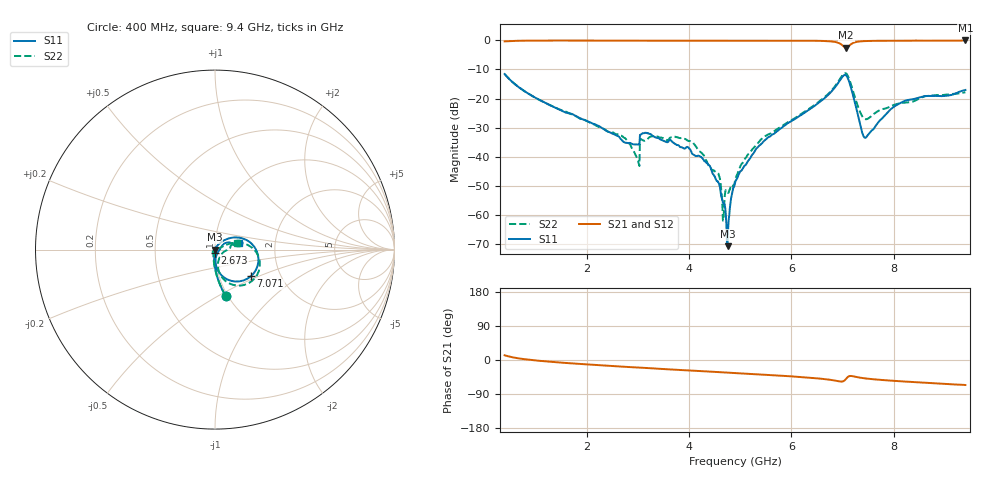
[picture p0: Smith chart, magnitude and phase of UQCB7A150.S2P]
!  Part Number  UQCB7A150	Mounting Orientation: Vertical
!  Description: RF capacitors
!  Application: Coupling, Bypass, Tuning, DC Block
!  Filters, Matching
# GHZ S DB R 50
! Freq  |S11|  S11 Ph  |S21|  S21 Ph  |S12|  S12 Ph  |S22|  S22 Ph
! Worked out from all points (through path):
!   801 points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, 400 MHz to 9.4 GHz, reference 50 ohm
!   highest |S21| = -0.02 dB at 9.4 GHz (marker M1); lowest = -2.5 dB at 7.071 GHz (marker M2)
!   group delay of S21, straight-line fit = 21.3 ps
!   lowest |S11| = -70.7 dB at 4.754 GHz (marker M3), VSWR 1.00, Z = 50 - j0.00383 ohm
!   |S11| at or under -10 dB: start of sweep to end of sweep
!   |S22| runs from -62.0 to -11.2 dB; largest |S21 - S12| = 0.0031
!   S11 on the Smith chart (normalised r, x): 400 MHz: 0.98, -0.54; 2.673 GHz: 1.00, -0.04; 7.071 GHz: 1.42, -0.45; 9.4 GHz: 1.31, +0.10
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0.4  -11.57 -77.1  -0.33 12.5  -0.32 12.5  -11.55 -77.1
1.908  -27.04 -94.8  -0.06 -10.7  -0.04 -10.7  -26.93 -101.3
2.673  -33.98 -89.0  -0.06 -17.2  -0.05 -17.2  -32.76 -109.5
2.988  -35.78 -68.2  -0.08 -19.9  -0.07 -19.9  -40.50 -126.9
3.089  -31.99 -85.2  -0.11 -20.7  -0.09 -20.7  -34.23 -112.5
3.404  -33.59 -99.4  -0.07 -23.0  -0.05 -23.1  -33.16 -112.1
4.045  -38.27 -117.7  -0.11 -27.9  -0.10 -28.0  -34.92 -135.3
4.383  -42.80 -129.3  -0.09 -30.4  -0.08 -30.5  -42.98 -140.8
4.574  -48.84 -165.8  -0.09 -32.0  -0.09 -32.1  -45.67 -129.6
4.664  -55.82 76.8  -0.10 -32.6  -0.10 -32.7  -61.97 -117.6
4.754  -70.74 -172.4  -0.09 -33.3  -0.08 -33.3  -52.12 -46.0
4.9  -49.05 79.0  -0.08 -34.5  -0.08 -34.5  -48.37 4.8
5.046  -44.21 70.1  -0.09 -35.7  -0.08 -35.7  -42.20 16.2
5.406  -35.70 65.6  -0.11 -38.5  -0.11 -38.5  -34.10 22.3
6.408  -23.10 46.3  -0.12 -47.3  -0.12 -47.4  -22.77 22.7
6.891  -15.23 19.8  -0.68 -55.3  -0.68 -55.4  -14.82 8.6
7.071  -12.08 -36.7  -2.54 -49.4  -2.55 -49.5  -11.37 -40.7
7.206  -18.94 -82.8  -0.89 -42.9  -0.90 -43.0  -17.48 -78.9
7.431  -33.42 -39.6  -0.24 -48.4  -0.25 -48.5  -26.99 -45.0
7.904  -24.31 33.0  -0.12 -54.0  -0.13 -54.1  -22.94 2.6
8.241  -20.63 24.7  -0.13 -57.0  -0.13 -57.1  -21.34 7.3
9.4  -17.04 15.7  -0.02 -66.0  -0.03 -66.1  -17.82 17.4
